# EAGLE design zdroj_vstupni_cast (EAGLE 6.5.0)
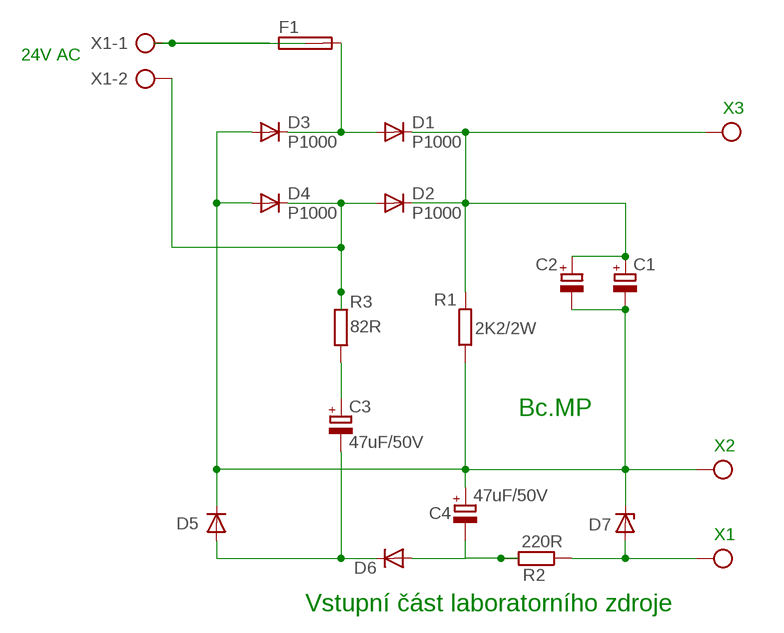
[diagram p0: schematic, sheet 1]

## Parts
C1  CPOL-EUE10-25  [EB25D]
C2  CPOL-EUE10-25  [EB25D]
C3  47uF/50V  CPOL-EUE2.5-7  [E2,5-7]
C4  47uF/50V  CPOL-EUE2.5-7  [E2,5-7]
D1  P1000  P600  [P6-15]
D2  P1000  P600  [P6-15]
D3  P1000  P600  [P6-15]
D4  P1000  P600  [P6-15]
D5  1N4148  1N4148DO35-7  [DO35-7]
D6  1N4148  1N4148DO35-7  [DO35-7]
D7  BZX83V005.6  [DO35Z10]
F1  SH22,5A  [SH22,5A]
R1  2K2/2W  R-EU_0411/15  [0411/15]
R2  220R  R-EU_0207/7  [0207/7]
R3  82R  R-EU_0207/7  [0207/7]
X1  AK500/2  [AK500/2]
X3-3  X-3-3  AK500/3  [AK500/3]

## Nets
N$1: D1.A D3.C F1.2
N$2: C1.- C2.- C4.+ D3.A D4.A D5.C D7.C R1.1 X3-3.2
N$3: F1.1 X1.1
N$6: C1.+ C2.+ D1.C D2.C R1.2 X3-3.3
N$7: D2.A D4.C R3.1 X1.2
N$8: C3.+ R3.2
N$9: C4.- D6.A R2.2
N$10: C3.- D5.A D6.C
N$11: D7.A R2.1 X3-3.1

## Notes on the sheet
- 24V | AC
- X3
- Bc.MP
- X2
- X1
- Vstupní část laboratorního zdroje

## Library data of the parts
C1-C4 = rcl:CPOL-EU: POLARIZED CAPACITOR, European symbol
D1-D4 = diode:P600: DIODE
D5 D6 = diode:1N4148: DIODE
D7 = zenerovy diody:BZX83V005.6: Zenerova dioda 0,5 W
F1 = fuse:SH22,5A: FUSE HOLDER; MPN: 0031.7701.11; OC_FARNELL: unknown; OC_NEWARK: 04F1224
R1-R3 = resistor:R-EU_: RESISTOR, European symbol
X1 = con-ptr500:AK500/2: CONNECTOR; OC_FARNELL: unknown; OC_NEWARK: unknown
X3-3 = con-ptr500:AK500/3: CONNECTOR; OC_FARNELL: unknown; OC_NEWARK: unknown

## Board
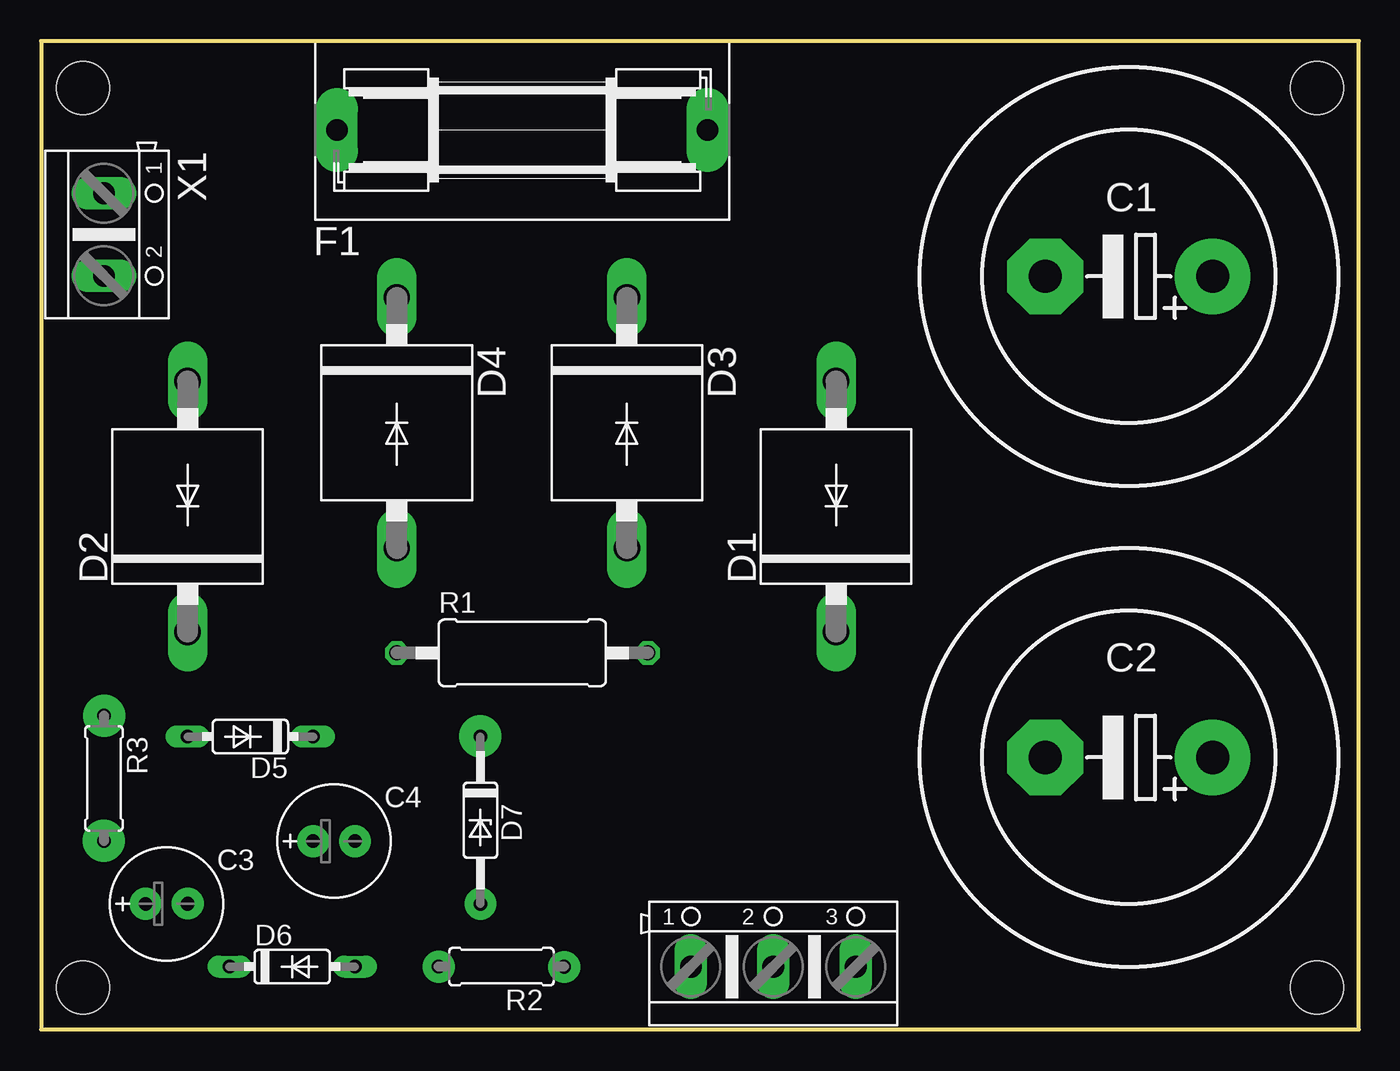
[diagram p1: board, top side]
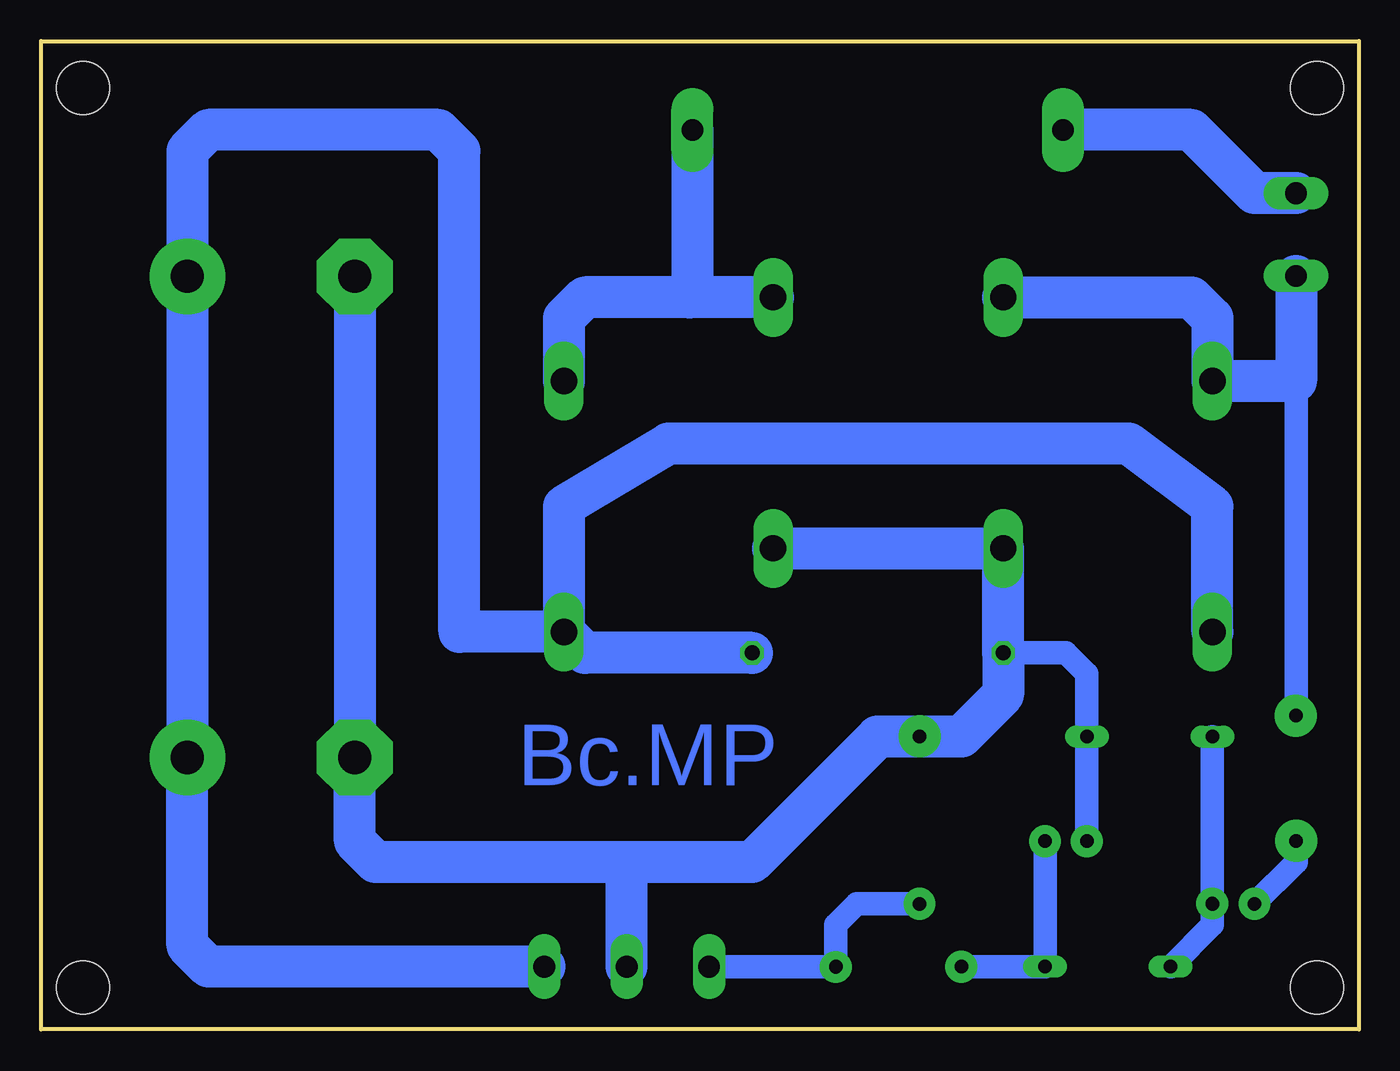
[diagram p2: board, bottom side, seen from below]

Size 80 x 60 mm. Coordinates in mm from the lower left corner, seen from the top.
Outline: 0,0 80,0 80,60 0,60 0,0
Copper layers (1*16): Top 0.035mm / dielectric 1.5mm / Bottom 0.035mm
Design rules "default": minimum track width 10mil, minimum drill 24mil, track to track 8mil, track to pad 8mil, pad to pad 8mil, via to via 8mil, smd to smd 8mil, copper to edge 40mil, drill to drill 8mil, minimum pad ring 10mil, minimum via ring 8mil, stop-mask expansion 4mil, vias tented up to drill 0mil, thermal gap 10mil
Holes 3.2 mm at 2.54,57.15 2.54,2.54 77.47,2.54 77.47,57.15

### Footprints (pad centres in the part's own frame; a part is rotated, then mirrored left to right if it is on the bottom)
EB25D = drill 2.007 pad 4.597: + -5.08,0 | drill 2.007 pad 4.597 octagon: - 5.08,0
E2,5-7 = drill 0.813 pad 1.6: + -1.27,0 | drill 0.813 pad 1.6 octagon: - 1.27,0
P6-15 = drill 1.6 long: A 7.62,0; C -7.62,0
DO35-7 = drill 0.813 long: A 3.81,0; C -3.81,0
DO35Z10 = drill 0.813 pad 1.676 octagon: A 5.08,0 | drill 0.813 pad 1.676: C -5.08,0
SH22,5A = drill 1.321 pad 2.54 long: 1 -11.252,0; 2 11.252,0
0411/15 = drill 0.914 octagon: 1 -7.62,0; 2 7.62,0
0207/7 = drill 0.813 octagon: 1 -3.81,0; 2 3.81,0
AK500/2 = drill 1.321 long: 1 -2.515,0; 2 2.515,0
AK500/3 = drill 1.321 long: 1 -5.004,0; 2 0,0; 3 5.004,0

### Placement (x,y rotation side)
C1  66.04,45.72 180 top
C2  66.04,16.51 180 top
C3  7.62,7.62 0 top
C4  17.78,11.43 0 top
D1  48.26,31.75 90 top
D2  8.89,31.75 90 top
D3  35.56,36.83 270 top
D4  21.59,36.83 270 top
D5  12.7,17.78 180 top
D6  15.24,3.81 0 top
D7  26.67,12.7 270 top
F1  29.21,54.61 0 top
R1  29.21,22.86 0 top
R2  27.94,3.81 180 top
R3  3.81,15.24 270 top
X1  3.81,48.26 270 top
X3-3  44.45,3.81 0 top

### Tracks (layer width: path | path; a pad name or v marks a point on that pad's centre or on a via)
N$1
  Bottom 0.813: 40.46,44.63 40.64,44.45
  Bottom 2.54: D3.C 40.64,44.45 46.99,44.45 48.26,43.18 D1.A | F1.2 40.46,44.63
N$2
  Bottom 1.422: R1.1 17.78,22.86 16.51,21.59 D5.C C4.+
  Bottom 2.54: C1.- C2.- 60.96,11.43 59.69,10.16 44.45,10.16 | D3.A D4.A R1.1 21.59,20.32 24.13,17.78 D7.C 29.21,17.78 36.83,10.16 44.45,10.16 | X3-3.2 44.45,10.16
N$3
  Bottom 2.54: X1.1 6.33,50.77 10.16,54.61 F1.1
N$4  (via drill 0.8 pad 2.54)
  other vias: 3.82,19.05
N$5  (via drill 0.8 pad 2.54)
  other vias: 3.8,11.45
N$6
  Bottom 2.54: D2.C 8.89,31.75 13.97,35.56 41.91,35.56 48.26,31.75 D1.C | D1.C 54.61,24.13 54.61,53.34 55.88,54.61 69.85,54.61 71.12,53.34 C1.+ C2.+ 71.12,5.08 69.85,3.81 X3-3.3 | R1.2 46.99,22.86 D1.C
N$7
  Bottom 1.422: 3.81,39.37 R3.1
  Bottom 2.54: X1.2 3.81,39.37 D2.A 8.89,43.18 10.16,44.45 D4.C
N$8
  Bottom 1.422: R3.2 3.81,10.16 C3.+
N$9
  Bottom 1.422: R2.2 D6.A C4.-
N$10
  Bottom 1.422: D5.A C3.- 8.89,6.35 D6.C
N$11
  Bottom 1.422: D7.A 30.48,7.62 31.75,6.35 R2.1 X3-3.1
N$12  (via drill 0.8 pad 2.54)
  other vias: 26.65,17.8
N$13  (via drill 0.8 pad 1.93)
  other vias: 6.33,7.64
N$14  (via drill 0.8 pad 1.93)
  other vias: 8.89,7.65
N$15  (via drill 0.8 pad 1.93)
  other vias: 16.51,11.43
N$16  (via drill 0.8 pad 1.93)
  other vias: 19.06,11.43
N$17  (via drill 0.8 pad 1.93)
  other vias: 24.13,3.8
N$18  (via drill 0.8 pad 1.93)
  other vias: 31.75,3.79
N$19  (via drill 0.8 pad 1.93)
  other vias: 26.68,7.62

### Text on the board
Bottom: Bc.MP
